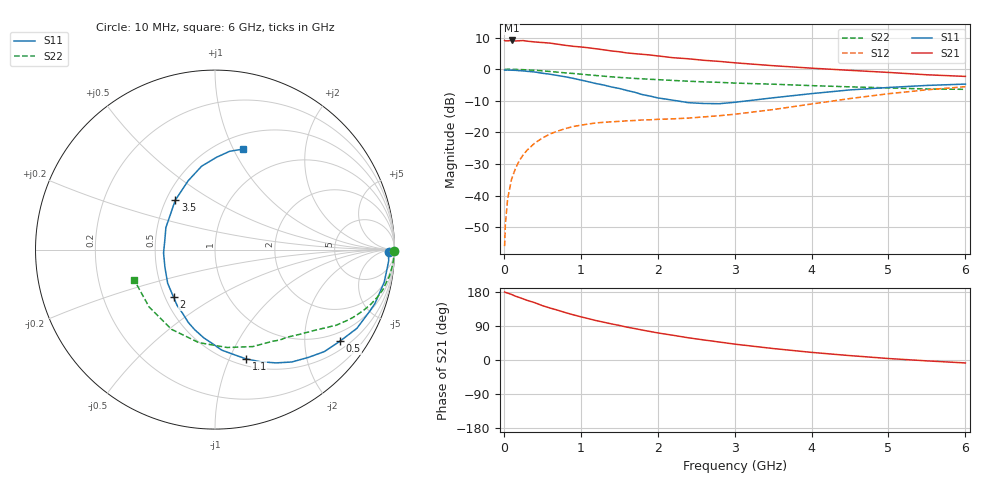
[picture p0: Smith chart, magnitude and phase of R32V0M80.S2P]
! SIEMENS Small Signal Semiconductors
! BFR181
! Si NPN RF Bipolar Junction Transistor in SOT23
! VCE = 2 V  IC = 0.8 mA
! Common Emitter S-Parameters:  May  1996
# GHz  S  MA  R  50
!  f  S11  S21  S12  S22
! GHz  MAG  ANG  MAG  ANG  MAG  ANG  MAG  ANG
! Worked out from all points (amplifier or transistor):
!   36 points, 10 MHz to 6 GHz, reference 50 ohm
!   highest |S21| = 9.1 dB at 100 MHz (marker M1)
!   |S21| within 3 dB of that: start of sweep to 1.311 GHz
!   unconditionally stable (mu >= 1): 2.109 GHz to 3.785 GHz
!   at 250 MHz: K = 0.14, MSG = 18.1 dB, |S12| = -27.1 dB
!   at 1.4 GHz: K = 0.72, MSG = 11.2 dB, |S12| = -16.6 dB
!   at 6 GHz: K = 0.89, MSG = 1.6 dB, |S12| = -5.5 dB
!   S11 on the Smith chart (normalised r, x): 10 MHz: 53, -23; 500 MHz: 0.72, -2.90; 1.1 GHz: 0.57, -1.15; 2 GHz: 0.55, -0.34; 3.5 GHz: 0.56, +0.35; 6 GHz: 0.65, +1.09
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0.01  0.9688 -0.8  2.842 179.5  0.0016 93.1  0.9994 -0.4
0.02  0.9655 -1.4  2.804 178.4  0.0035 91.7  0.9905 -0.7
0.05  0.9699 -3.6  2.804 176.5  0.0091 88.0  0.9982 -1.7
0.1  0.9634 -7.3  2.844 173.1  0.0182 85.1  0.9957 -3.4
0.15  0.9597 -11.0  2.793 168.5  0.0268 82.5  0.9919 -5.3
0.25  0.9401 -18.7  2.833 161.4  0.044 77.2  0.9829 -8.6
0.4  0.9043 -29.0  2.694 151.4  0.0678 70.9  0.9619 -13.4
0.5  0.8634 -36.2  2.638 143.5  0.0816 66.7  0.9419 -16.4
0.6  0.8332 -43.0  2.582 137.2  0.0947 62.5  0.9203 -19.3
0.8  0.7581 -55.7  2.38 125.1  0.1153 55.5  0.8752 -24.2
1  0.6743 -67.9  2.245 114.1  0.1304 50.0  0.8343 -28.3
1.1  0.6327 -74.2  2.178 109.1  0.1362 47.8  0.8135 -30.2
1.4  0.5235 -91.6  1.941 95.2  0.1474 42.7  0.7575 -35.1
1.6  0.461 -104.1  1.806 86.7  0.1529 40.9  0.7292 -37.6
2  0.3521 -130.9  1.621 71.5  0.1614 39.9  0.6837 -42.7
2.2  0.3236 -144.6  1.518 65.2  0.1643 40.6  0.6639 -45.5
2.4  0.2956 -160.8  1.46 58.6  0.169 42.2  0.6457 -48.2
2.8  0.285 168.3  1.328 47.5  0.1841 45.3  0.6198 -54.4
3.5  0.3532 128.8  1.136 30.3  0.2303 49.8  0.5796 -68.8
4.5  0.4708 99.1  0.959 11.6  0.3437 47.1  0.5261 -99.8
5.5  0.5539 81.5  0.816 -2.3  0.4727 34.5  0.4868 -138.9
6  0.5814 74.4  0.769 -7.8  0.529 26.4  0.4808 -159.3
